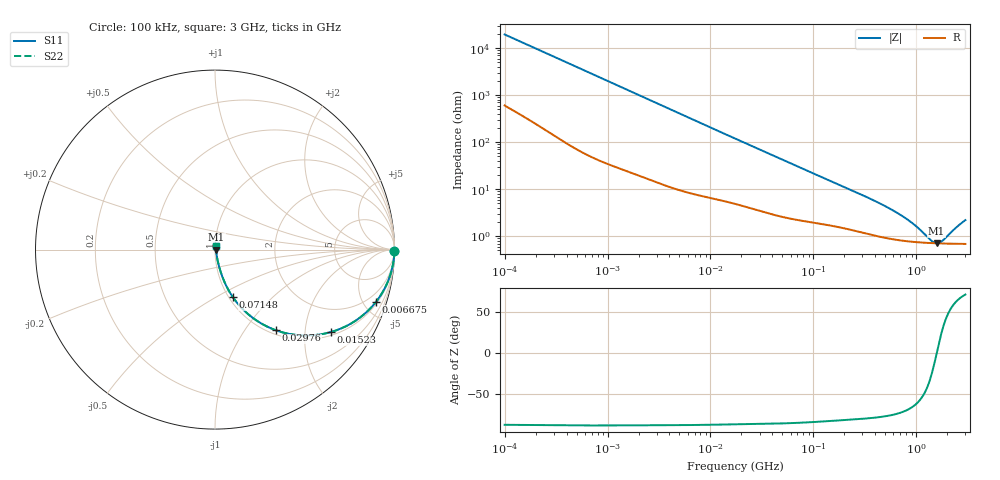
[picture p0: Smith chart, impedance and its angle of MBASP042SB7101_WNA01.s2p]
! MBASP042SB7101_WNA01  S-PARAMETER MODEL  ( Standard Model )
! Model Generated by TAIYO YUDEN Corporation (https://www.yuden.co.jp/en/)
! Version 1.0
! TAIYO YUDEN Control No. 250312
! Copyright(c) 2025 TAIYO YUDEN CO.,LTD. All Rights Reserved.
! Product Description (link to TY-COMPAS)
! https://ds.yuden.co.jp/TYCOMPAS/or/detail?pn=MBASP042SB7101KWNA01&u=M
! Products Name : Multilayer Ceramic Capacitors
! Characteristics :
!  Capacitance : 100 [pF] , Rated Voltage : 2.5 [V] , TCC : X7R
!  Case Size : 0.4 x 0.2 / 0.016 x 0.008 [mm/inch] , Thickness : 0.2 / 0.008 [mm/inch]
!  (Conditions: Temperature = 25 [degC] , DC Bias Voltage = 0 [V])
! External Node Assignments :
!  1  o---| |---o  2
! GND o---------o GND
! Frequency Range : 100kHz  -  3GHz  [ 401 STEP ]
# MHZ S RI R 50
! Freq[MHz].  S11 Real  S11 Imag  S21 Real  S21 Imag  S12 Real  S12 Imag  S22 Real  S22 Imag
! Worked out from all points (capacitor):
!   401 points, 100 kHz to 3 GHz, reference 50 ohm
!   read as one part in series: C = 81.3 pF near 105.3 kHz
!   lowest |Z| = 710 mohm at 1.575 GHz (marker M1)
!   series resonance near 1.581 GHz, so ESL is about 120 pH
!   S11 on the Smith chart (normalised r, x): 100 kHz: open; 6.675 MHz: 1.16, -6.11; 15.23 MHz: 1.11, -2.72; 29.76 MHz: 1.07, -1.41; 71.48 MHz: 1.04, -0.60; 3 GHz: 1.01, +0.04
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0.1  0.9998 -0.00513  0.000185 0.00513  0.000185 0.00513  0.9998 -0.00513
0.562235  0.9987 -0.0282  0.00128 0.0282  0.00128 0.0282  0.9987 -0.0282
1.497078  0.9931 -0.0739  0.00687 0.0739  0.00687 0.0739  0.9931 -0.0739
3.161081  0.9732 -0.1514  0.0268 0.1514  0.0268 0.1514  0.9732 -0.1514
6.674626  0.8973 -0.2908  0.1027 0.2908  0.1027 0.2908  0.8973 -0.2908
10.08119  0.7982 -0.3857  0.2018 0.3857  0.2018 0.3857  0.7982 -0.3857
15.22638  0.6435 -0.46  0.3565 0.46  0.3565 0.46  0.6435 -0.46
17.7727  0.5743 -0.4742  0.4257 0.4742  0.4257 0.4742  0.5743 -0.4742
22.99754  0.4545 -0.4758  0.5455 0.4758  0.5455 0.4758  0.4545 -0.4758
29.75839  0.3407 -0.4499  0.6593 0.4499  0.6593 0.4499  0.3407 -0.4499
46.11977  0.1889 -0.3633  0.8111 0.3633  0.8111 0.3633  0.1889 -0.3633
71.47675  0.0989 -0.264  0.9011 0.264  0.9011 0.264  0.0989 -0.264
97.38194  0.0635 -0.2035  0.9365 0.2035  0.9365 0.2035  0.0635 -0.2035
205.6221  0.0253 -0.1034  0.9747 0.1034  0.9747 0.1034  0.0253 -0.1034
547.5153  0.0103 -0.0375  0.9897 0.0375  0.9897 0.0375  0.0103 -0.0375
848.5431  0.00811 -0.0198  0.9919 0.0198  0.9919 0.0198  0.00811 -0.0198
1042.837  0.00757 -0.0129  0.9924 0.0129  0.9924 0.0129  0.00757 -0.0129
1384.641  0.00715 -0.004  0.9929 0.004  0.9929 0.004  0.00715 -0.004
1575.075  0.00705 -0.000108  0.9929 0.000108  0.9929 0.000108  0.00705 -0.000108
1791.7  0.007 0.00379  0.993 -0.00379  0.993 -0.00379  0.007 0.00379
2504.792  0.00708 0.0144  0.9929 -0.0144  0.9929 -0.0144  0.00708 0.0144
3000  0.00727 0.0207  0.9927 -0.0207  0.9927 -0.0207  0.00727 0.0207
